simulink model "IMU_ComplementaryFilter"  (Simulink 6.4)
settings: Solver=FixedStepDiscrete  StartTime=0.0  StopTime=10.0  FixedStep=0.001  RelTol=1e-3
undefined symbols (not defined in the file or in its folder): bits, float, gaind, hex2dec, polesd, tustin, zerosd
libraries: dsPICdrivers x31, simulink x13

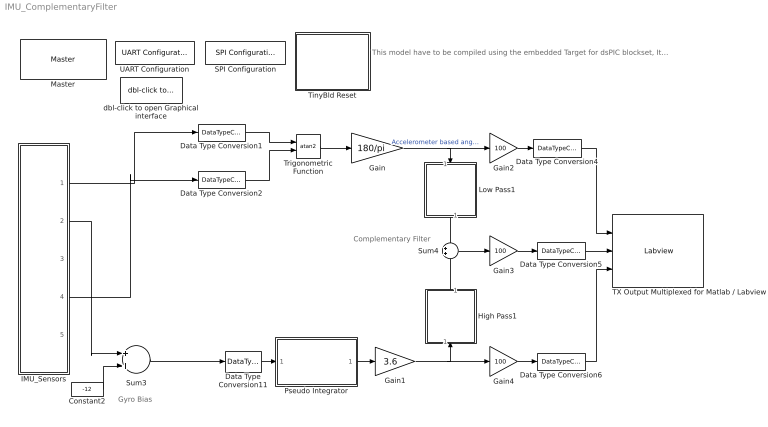
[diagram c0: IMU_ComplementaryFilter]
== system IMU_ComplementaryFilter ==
  note: Gyro Bias
  note: Complementary Filter
  note: This model have to be compiled using the embedded Target for dsPIC blockset, It run on the dsPIC 30f4012 but can be addapted for others MCU.
  Constant2 : Constant  Value=-12  OutDataType=sfix(16)  OutScaling=2^0  SampleTime=-1
  Data Type Conversion1 : DataTypeConversion  OutDataTypeMode=single  OutDataType=sfix(16)  OutScaling="[ (80/(2048*2^4))  0]"
  Data Type Conversion11 : DataTypeConversion  OutDataTypeMode=double  OutDataType=sfix(16)  OutScaling="[ (80/(2048*2^4))  0]"
  Data Type Conversion2 : DataTypeConversion  OutDataTypeMode=single  OutDataType=sfix(16)  OutScaling="[ (80/(2048*2^4))  0]"
  Data Type Conversion4 : DataTypeConversion  OutDataTypeMode=int16  OutDataType=sfix(16)  OutScaling="[ (80/(2048*2^4))  0]"
  Data Type Conversion5 : DataTypeConversion  OutDataTypeMode=int16  OutDataType=sfix(16)  OutScaling="[ (80/(2048*2^4))  0]"
  Data Type Conversion6 : DataTypeConversion  OutDataTypeMode=int16  OutDataType=sfix(16)  OutScaling="[ (80/(2048*2^4))  0]"
  Gain : Gain  Gain=180/pi  ParameterDataType=sfix(16)  ParameterScaling=2^0  OutDataTypeMode=Specify via dialog  OutDataType=float('double')  OutScaling=2^0
  Gain1 : Gain  Gain=3.6  ParameterDataType=sfix(16)  ParameterScaling=2^0  OutDataTypeMode=Specify via dialog  OutDataType=float('double')  OutScaling=2^0
  Gain2 : Gain  Gain=100  ParameterDataType=sfix(16)  ParameterScaling=2^0  OutDataTypeMode=Specify via dialog  OutDataType=float('double')  OutScaling=2^0
  Gain3 : Gain  Gain=100  ParameterDataType=sfix(16)  ParameterScaling=2^0  OutDataTypeMode=Specify via dialog  OutDataType=float('double')  OutScaling=2^0
  Gain4 : Gain  Gain=100  ParameterDataType=sfix(16)  ParameterScaling=2^0  OutDataTypeMode=Specify via dialog  OutDataType=float('double')  OutScaling=2^0
  High Pass1 : Subsystem  Orientation=up  mask(DiscretizedZeroPole){Zeros=[0], Poles=[-.5], Gain=1, AbsTol=auto, SampleTime=.001, method=tustin, Wc=1}
      mask prompts: Zeros "Zeros (enter in s-main:)"; Poles "Poles (enter in s-domain:)"; Gain "Gain (enter in s-domain:)"; AbsTol "Absolute tolerance:"; SampleTime "Sample time:"; Wc "Critical Frequency (Hz):"
      mask help: Continuous mask uses c2d to transform parameters onto the Discrete Zero-Pole block inside.
      mask init:
      | st=SampleTime;
      | if length(st)>1
      |     st=SampleTime(1);
      | end
      | if(st>0)
      |     [zerosd,polesd,gaind] = sldiscutil('disczpk', {st,method,Wc,Zeros,Poles,Gain});
      | end	
      | s = get_param(gcb,'maskvalues');
      | zeross = s{1};
      | poless = s{2};
      | gainss = s{3};
      | %zerosc = eval(zeross);
      | %polesc = eval(poless);
      | %gainsc = eval(gainss);
      | sldiscutil('initzpkmask', st);
      | if(st==0)
      | set_param([gcb '/Zero Pole'], 'AbsoluteTolerance', AbsTol);
      | end
  IMU_Sensors : Subsystem
  Low Pass1 : Subsystem  Orientation=down  mask(DiscretizedZeroPole){Zeros=[], Poles=[-.5], Gain=.5, AbsTol=auto, SampleTime=.001, method=tustin, Wc=1}
      mask prompts: Zeros "Zeros (enter in s-main:)"; Poles "Poles (enter in s-domain:)"; Gain "Gain (enter in s-domain:)"; AbsTol "Absolute tolerance:"; SampleTime "Sample time:"; Wc "Critical Frequency (Hz):"
      mask help: Continuous mask uses c2d to transform parameters onto the Discrete Zero-Pole block inside.
      mask init:
      | st=SampleTime;
      | if length(st)>1
      |     st=SampleTime(1);
      | end
      | if(st>0)
      |     [zerosd,polesd,gaind] = sldiscutil('disczpk', {st,method,Wc,Zeros,Poles,Gain});
      | end	
      | s = get_param(gcb,'maskvalues');
      | zeross = s{1};
      | poless = s{2};
      | gainss = s{3};
      | %zerosc = eval(zeross);
      | %polesc = eval(poless);
      | %gainsc = eval(gainss);
      | sldiscutil('initzpkmask', st);
      | if(st==0)
      | set_param([gcb '/Zero Pole'], 'AbsoluteTolerance', AbsTol);
      | end
  Master : dsPICdrivers/Master  Tag=dsPIC_MASTER  Priority=1  TimeStepType=Timer1  picType=30f4012  fcy=20e6  Quartz_33f=5e6  PLLActive_33f=off  fcyDesired_33f=0  tmr1="[1  19999  0]"  tmr1Info="Time Step : 0.001  ;   Error : 0%  PR1=19999"  tmr2345="[0  0  0  0]"  tmr2345cfg=[-1 -1 -1 -1]  IOautoConf=on  typePort="[ 0   0   0   0   0   0   0   0   0   0   0   0   0   0   0   0   0   0   0   0   0   0   0   0   0   0   0   0   0   0   0   0   0   0   0   0   0   0   0   0   0   0   0   0   0   5   4   0   0   0   0   0   0   0   0   0   0   0   0   0   0   0   0   0   0   0   0  10   0  10   0   0  17   0   0   0   0   0   0   0   0   0  14  15   0   0   0   0   0   0   0   0   0   0   0   0   0   0   0   0 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"  TRIS="[ 65535  65535  65535  65535  65495  65535  65535 ]"  ADPCFG=0  MasterBusyPort=None  MasterOverloadPort=None  FOSC=XT_PLL8  TempProtection_33f=TEMP_ON  FPBOR=PBOR_OFF  PWRT=PWRT_4  MCLR=MCLR_DIS  PowerSave=off
  Pseudo Integrator : Subsystem  mask(DiscretizedZeroPole){Zeros=[0 -314], Poles=[-.03 -.03], Gain=(1/314), AbsTol=auto, SampleTime=.001, method=tustin, Wc=1}
      mask prompts: Zeros "Zeros (enter in s-main:)"; Poles "Poles (enter in s-domain:)"; Gain "Gain (enter in s-domain:)"; AbsTol "Absolute tolerance:"; SampleTime "Sample time:"; Wc "Critical Frequency (Hz):"
      mask help: Continuous mask uses c2d to transform parameters onto the Discrete Zero-Pole block inside.
      mask init:
      | st=SampleTime;
      | if length(st)>1
      |     st=SampleTime(1);
      | end
      | if(st>0)
      |     [zerosd,polesd,gaind] = sldiscutil('disczpk', {st,method,Wc,Zeros,Poles,Gain});
      | end	
      | s = get_param(gcb,'maskvalues');
      | zeross = s{1};
      | poless = s{2};
      | gainss = s{3};
      | %zerosc = eval(zeross);
      | %polesc = eval(poless);
      | %gainsc = eval(gainss);
      | sldiscutil('initzpkmask', st);
      | if(st==0)
      | set_param([gcb '/Zero Pole'], 'AbsoluteTolerance', AbsTol);
      | end
  SPI Configuration : dsPICdrivers/SPI PORT/SPI Configuration  Tag=dsPIC_config_SPI  Priority=2  ConfigurationTime=At boot time (only once)  OrderingInOutPopup=None  SampleTime=-1  Frame_Enable=0  Frame_Sync=0  SPI=1  MODE=MASTER  USER_SCALER=12  StartEnable=Enable  SDO_EN=on  DATA_LENGTH=16 bits  SS_EN=off  SMP=Middle of bit  CKP=high  CKE=Idle to Active  Status="Mode 1  -    Fsck= Not Available"
  Sum3 : Sum  OutDataType=sfix(16)  OutScaling=2^0
  Sum4 : Sum  OutDataType=sfix(16)  OutScaling=2^0
  TX Output Multiplexed for Matlab / Labview : dsPICdrivers/Serial PORT/TX Output Multiplexed for Matlab // Labview  Tag=dsPIC_TX_Multiplexed  Priority=5  UART=1  CleverSpreadingChk=on  CleverSpreading=1  CHANNEL=[0 1 2 ]  BUFFERSIZE=16  CHANNELBLOCKED=[]  CHANNELBLOCKED_BITEWISE=0  Status=OK
  TinyBld Reset : Subsystem  AncestorBlock=dsPICdrivers/OTHERS/TinyBld Reset
  Trigonometric Function : Trigonometry  Operator=atan2  OutputSignalType=real
  UART Configuration : dsPICdrivers/Serial PORT/UART Configuration  Tag=dsPIC_config_UART  Priority=2  UART=1  proposed_BAUD=115200  ALT_TX_RX=on  TXInterruptPri=1  InterruptTxWhen=on TxBUF becoming empty  TXEN=on  RXInterruptPri=1  BAUD=115200  UxBRG=10  Info="UxBRG = 10   ||  Real Baud : 113636   ||  % error : -1.3573  ||  max 11.3636 Bytes / Step"  RealBaud=0
  dbl-click to open Graphical interface : dsPICdrivers/Serial PORT/dbl-click to open Graphical interface  SystemSampleTime=-1
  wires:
  Trigonometric Function/1 -> Gain/1
  Constant2/1 -> Sum3/2
  Low Pass1/1(Out1) -> Sum4/1
  High Pass1/1(Out1) -> Sum4/2
  Pseudo Integrator/1(Out1) -> Gain1/1
  Gain1/1 -> High Pass1/1(In1), Gain4/1
  Gain/1 -> Low Pass1/1(In1), Gain2/1  "Accelerometer based angle estimation"
  Sum4/1 -> Gain3/1
  Data Type Conversion2/1 -> Trigonometric Function/2
  Data Type Conversion1/1 -> Trigonometric Function/1
  Data Type Conversion11/1 -> Pseudo Integrator/1(In1)
  Sum3/1 -> Data Type Conversion11/1
  IMU_Sensors/1(AccelX) -> Data Type Conversion1/1
  IMU_Sensors/4(AccelZ) -> Data Type Conversion2/1
  IMU_Sensors/2(GyroY) -> Sum3/1
  Data Type Conversion4/1 -> TX Output Multiplexed for Matlab / Labview/1
  Gain2/1 -> Data Type Conversion4/1
  Gain3/1 -> Data Type Conversion5/1
  Gain4/1 -> Data Type Conversion6/1
  Data Type Conversion5/1 -> TX Output Multiplexed for Matlab / Labview/2
  Data Type Conversion6/1 -> TX Output Multiplexed for Matlab / Labview/3

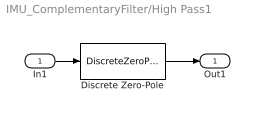
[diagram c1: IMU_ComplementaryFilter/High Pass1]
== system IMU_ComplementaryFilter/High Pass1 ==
  In1 : Inport  OutDataType=sfix(16)  OutScaling=2^0
  Discrete Zero-Pole : DiscreteZeroPole  Zeros=zerosd  Poles=polesd  Gain=gaind  SampleTime=SampleTime
  Out1 : Outport  OutDataType=sfix(16)  OutScaling=2^0
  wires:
  Discrete Zero-Pole/1 -> Out1/1
  In1/1 -> Discrete Zero-Pole/1

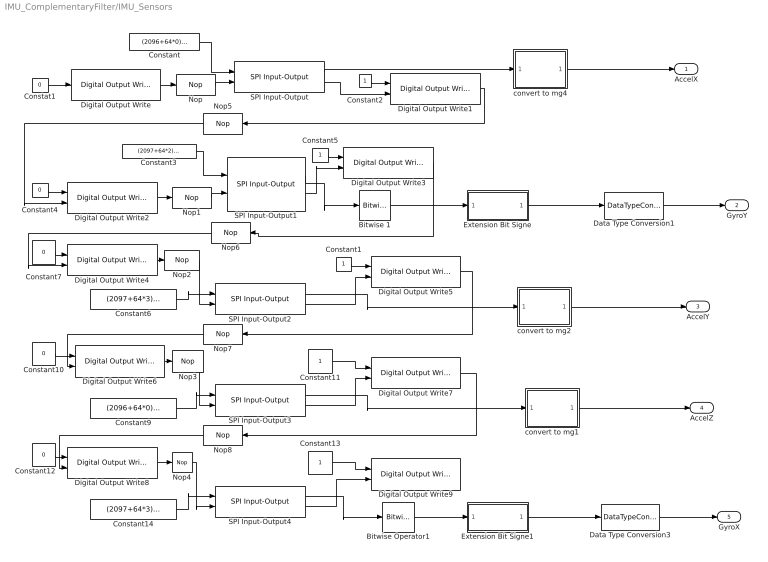
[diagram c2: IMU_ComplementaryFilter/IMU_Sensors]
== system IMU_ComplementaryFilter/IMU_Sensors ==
  Bitwise Operator1 : simulink/Logic and Bit Operations/Bitwise Operator  logicop=AND  UseBitMask=on  BitMask=hex2dec('0FFF')  BitMaskRealWorld=Stored Integer
  Bitwise 1 : simulink/Logic and Bit Operations/Bitwise Operator  logicop=AND  UseBitMask=on  BitMask=hex2dec('0FFF')  BitMaskRealWorld=Stored Integer
  Constant : Constant  Value=(2096+64*0)*16  OutDataTypeMode=uint16  OutDataType=sfix(16)  OutScaling=2^0  SampleTime=-1
  Constant{1..2,5,11,13} (5 alike) : Constant  OutDataTypeMode=boolean  OutDataType=sfix(16)  OutScaling=2^0  SampleTime=-1
  Constant{4,7,10,12} (4 alike) : Constant  Value=0  OutDataTypeMode=boolean  OutDataType=sfix(16)  OutScaling=2^0  SampleTime=-1
  Constant14 : Constant  Value=(2097+64*3)*16  OutDataTypeMode=uint16  OutDataType=sfix(16)  OutScaling=2^0  SampleTime=-1
  Constant3 : Constant  Value=(2097+64*2)*16  VectorParams1D=off  OutDataTypeMode=uint16  OutDataType=sfix(16)  OutScaling=2^0  SampleTime=-1
  Constant6 : Constant  Value=(2097+64*3)*16  OutDataTypeMode=uint16  OutDataType=sfix(16)  OutScaling=2^0  SampleTime=-1
  Constant9 : Constant  Value=(2096+64*0)*16  OutDataTypeMode=uint16  OutDataType=sfix(16)  OutScaling=2^0  SampleTime=-1
  Constat1 : Constant  Value=0  OutDataTypeMode=boolean  OutDataType=sfix(16)  OutScaling=2^0  SampleTime=-1
  Data Type Conversion1 : DataTypeConversion  OutDataTypeMode=Specify via dialog  OutDataType=sfix(12)  OutScaling="[ (160/4096)  0]"  ConvertRealWorld=Stored Integer (SI)
  Data Type Conversion3 : DataTypeConversion  OutDataTypeMode=Specify via dialog  OutDataType=sfix(12)  OutScaling="[ (160/4096)  0]"  ConvertRealWorld=Stored Integer (SI)
  Digital Output Write : dsPICdrivers/Digital I//O/Digital Output Write  Tag=dsPIC_Digital_Output  Priority=5  PORT=E  Pin=5  Simultaneous=off  OrderingInOutPopup=Output
  Digital Output Write{1..5} (5 alike) : dsPICdrivers/Digital I//O/Digital Output Write  Tag=dsPIC_Digital_Output  Priority=5  PORT=E  Pin=5  Simultaneous=off  OrderingInOutPopup=Input & Output
  Digital Output Write6 : dsPICdrivers/Digital I//O/Digital Output Write  Tag=dsPIC_Digital_Output  Priority=5  PORT=E  Pin=3  Simultaneous=off  OrderingInOutPopup=Input & Output
  Digital Output Write7 : dsPICdrivers/Digital I//O/Digital Output Write  Tag=dsPIC_Digital_Output  Priority=5  PORT=E  Pin=3  Simultaneous=off  OrderingInOutPopup=Input & Output
  Digital Output Write8 : dsPICdrivers/Digital I//O/Digital Output Write  Tag=dsPIC_Digital_Output  Priority=5  PORT=E  Pin=3  Simultaneous=off  OrderingInOutPopup=Input & Output
  Digital Output Write9 : dsPICdrivers/Digital I//O/Digital Output Write  Tag=dsPIC_Digital_Output  Priority=5  PORT=E  Pin=3  Simultaneous=off  OrderingInOutPopup=Input
  Extension Bit Signe : Subsystem  TreatAsAtomicUnit=on
  Extension Bit Signe1 : Subsystem  TreatAsAtomicUnit=on
  Nop{,1..4} (5 alike) : dsPICdrivers/OTHERS/Nop  Tag=dsPIC_Reset  NbrNop=5
  Nop{5..8} (4 alike) : dsPICdrivers/OTHERS/Nop  Tag=dsPIC_Reset  Orientation=left  NbrNop=5
  SPI Input-Output{,1..4} (5 alike) : dsPICdrivers/SPI PORT/SPI Input-Output  Tag=dsPIC_SPI  SPI=1  INPUT=on  RESET_INPUT=off  OUTPUT=on  SPECIAL_SPI=Always Enable  DATA_LENGTH=16 bits  WAIT_INPUTDATA=on  OrderingInOutPopup=Input & Output  SampleTime=-1
  convert to mg1 : Subsystem  TreatAsAtomicUnit=on
  convert to mg2 : Subsystem  TreatAsAtomicUnit=on
  convert to mg4 : Subsystem  TreatAsAtomicUnit=on
  AccelX : Outport  OutDataType=sfix(16)  OutScaling=2^0
  GyroY : Outport  Port=2  OutDataType=sfix(16)  OutScaling=2^0
  AccelY : Outport  Port=3  OutDataType=sfix(16)  OutScaling=2^0
  AccelZ : Outport  Port=4  OutDataType=sfix(16)  OutScaling=2^0
  GyroX : Outport  Port=5  OutDataType=sfix(16)  OutScaling=2^0
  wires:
  Extension Bit Signe1/1(Out1) -> Data Type Conversion3/1
  Extension Bit Signe/1(Out1) -> Data Type Conversion1/1
  Bitwise 1/1 -> Extension Bit Signe/1(In1)
  Digital Output Write3/1 -> Nop6/1
  convert to mg2/1(Out1) -> AccelY/1
  convert to mg1/1(Out1) -> AccelZ/1
  Data Type Conversion3/1 -> GyroX/1
  Bitwise Operator1/1 -> Extension Bit Signe1/1(In1)
  Nop8/1 -> Digital Output Write8/2
  Nop7/1 -> Digital Output Write6/2
  Nop6/1 -> Digital Output Write4/2
  Nop5/1 -> Digital Output Write2/2
  Nop4/1 -> SPI Input-Output4/2
  Nop3/1 -> SPI Input-Output3/2
  Nop2/1 -> SPI Input-Output2/2
  Nop1/1 -> SPI Input-Output1/2
  Nop/1 -> SPI Input-Output/2
  Data Type Conversion1/1 -> GyroY/1
  convert to mg4/1(Out1) -> AccelX/1
  SPI Input-Output4/2 -> Digital Output Write9/2
  SPI Input-Output4/1 -> Bitwise Operator1/1
  Digital Output Write8/1 -> Nop4/1
  Constant14/1 -> SPI Input-Output4/1
  SPI Input-Output3/2 -> Digital Output Write7/2
  SPI Input-Output3/1 -> convert to mg1/1(In1)
  Constant9/1 -> SPI Input-Output3/1
  Digital Output Write6/1 -> Nop3/1
  SPI Input-Output2/2 -> Digital Output Write5/2
  SPI Input-Output2/1 -> convert to mg2/1(In1)
  Constant6/1 -> SPI Input-Output2/1
  Digital Output Write4/1 -> Nop2/1
  Constant7/1 -> Digital Output Write4/1
  SPI Input-Output1/1 -> Bitwise 1/1
  SPI Input-Output1/2 -> Digital Output Write3/2
  Digital Output Write2/1 -> Nop1/1
  Constant3/1 -> SPI Input-Output1/1
  SPI Input-Output/1 -> convert to mg4/1(In1)
  SPI Input-Output/2 -> Digital Output Write1/2
  Constant/1 -> SPI Input-Output/1
  Digital Output Write/1 -> Nop/1
  Digital Output Write7/1 -> Nop8/1
  Constant12/1 -> Digital Output Write8/1
  Constant13/1 -> Digital Output Write9/1
  Digital Output Write5/1 -> Nop7/1
  Constant10/1 -> Digital Output Write6/1
  Constant11/1 -> Digital Output Write7/1
  Constant1/1 -> Digital Output Write5/1
  Digital Output Write1/1 -> Nop5/1
  Constant4/1 -> Digital Output Write2/1
  Constant5/1 -> Digital Output Write3/1
  Constat1/1 -> Digital Output Write/1
  Constant2/1 -> Digital Output Write1/1

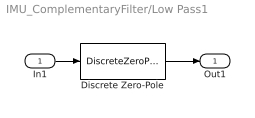
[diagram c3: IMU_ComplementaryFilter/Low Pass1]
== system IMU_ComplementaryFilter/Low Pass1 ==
  In1 : Inport  OutDataType=sfix(16)  OutScaling=2^0
  Discrete Zero-Pole : DiscreteZeroPole  Zeros=zerosd  Poles=polesd  Gain=gaind  SampleTime=SampleTime
  Out1 : Outport  OutDataType=sfix(16)  OutScaling=2^0
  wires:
  In1/1 -> Discrete Zero-Pole/1
  Discrete Zero-Pole/1 -> Out1/1

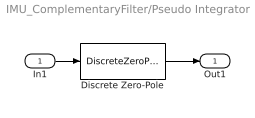
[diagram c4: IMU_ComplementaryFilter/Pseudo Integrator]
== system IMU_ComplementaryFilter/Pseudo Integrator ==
  In1 : Inport  OutDataType=sfix(16)  OutScaling=2^0
  Discrete Zero-Pole : DiscreteZeroPole  Zeros=zerosd  Poles=polesd  Gain=gaind  SampleTime=SampleTime
  Out1 : Outport  OutDataType=sfix(16)  OutScaling=2^0
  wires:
  Discrete Zero-Pole/1 -> Out1/1
  In1/1 -> Discrete Zero-Pole/1

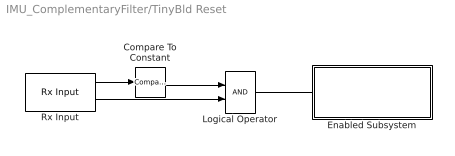
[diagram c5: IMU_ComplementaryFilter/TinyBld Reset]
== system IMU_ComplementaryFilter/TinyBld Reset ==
  Compare To Constant : simulink/Logic and Bit Operations/Compare To Constant  SystemSampleTime=-1  relop===  const=55  LogicOutDataTypeMode=boolean  ZeroCross=off
  Enabled Subsystem : Subsystem  Orientation=up  TreatAsAtomicUnit=on
  Logical Operator : Logic  AllPortsSameDT=off  OutDataTypeMode=boolean
  Rx Input : dsPICdrivers/Serial PORT/Rx Input  Tag=dsPIC_RX  Priority=5  UART=1  SampleTime=.01  BlockingFctChk=off  OutputDefault=0  IsPresentFlagChk=on
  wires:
  Rx Input/1 -> Compare To Constant/1
  Compare To Constant/1 -> Logical Operator/1
  Rx Input/2 -> Logical Operator/2
  Logical Operator/1 -> Enabled Subsystem/Enable

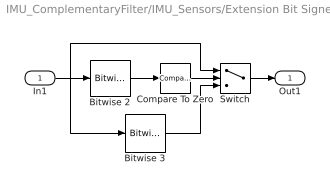
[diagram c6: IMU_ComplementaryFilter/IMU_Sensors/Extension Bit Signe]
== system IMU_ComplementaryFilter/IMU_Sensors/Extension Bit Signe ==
  In1 : Inport  OutDataType=sfix(16)  OutScaling=2^0
  Bitwise 2 : simulink/Logic and Bit Operations/Bitwise Operator  logicop=AND  UseBitMask=on  BitMask=2^11  BitMaskRealWorld=Stored Integer
  Bitwise 3 : simulink/Logic and Bit Operations/Bitwise Operator  logicop=OR  UseBitMask=on  BitMask=hex2dec('F000')  BitMaskRealWorld=Stored Integer
  Compare To Zero : simulink/Logic and Bit Operations/Compare To Zero  SystemSampleTime=-1  relop===  LogicOutDataTypeMode=boolean  ZeroCross=off
  Switch : Switch  Criteria=u2 ~= 0
  Out1 : Outport  OutDataType=sfix(16)  OutScaling=2^0
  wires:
  Switch/1 -> Out1/1
  Bitwise 3/1 -> Switch/3
  Compare To Zero/1 -> Switch/2
  Bitwise 2/1 -> Compare To Zero/1
  In1/1 -> Bitwise 2/1, Switch/1, Bitwise 3/1

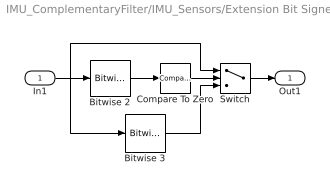
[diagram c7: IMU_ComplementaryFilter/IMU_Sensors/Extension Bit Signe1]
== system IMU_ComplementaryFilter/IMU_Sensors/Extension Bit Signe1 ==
  In1 : Inport  OutDataType=sfix(16)  OutScaling=2^0
  Bitwise 2 : simulink/Logic and Bit Operations/Bitwise Operator  logicop=AND  UseBitMask=on  BitMask=2^11  BitMaskRealWorld=Stored Integer
  Bitwise 3 : simulink/Logic and Bit Operations/Bitwise Operator  logicop=OR  UseBitMask=on  BitMask=hex2dec('F000')  BitMaskRealWorld=Stored Integer
  Compare To Zero : simulink/Logic and Bit Operations/Compare To Zero  SystemSampleTime=-1  relop===  LogicOutDataTypeMode=boolean  ZeroCross=off
  Switch : Switch  Criteria=u2 ~= 0
  Out1 : Outport  OutDataType=sfix(16)  OutScaling=2^0
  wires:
  In1/1 -> Bitwise 3/1, Switch/1, Bitwise 2/1
  Bitwise 2/1 -> Compare To Zero/1
  Compare To Zero/1 -> Switch/2
  Bitwise 3/1 -> Switch/3
  Switch/1 -> Out1/1

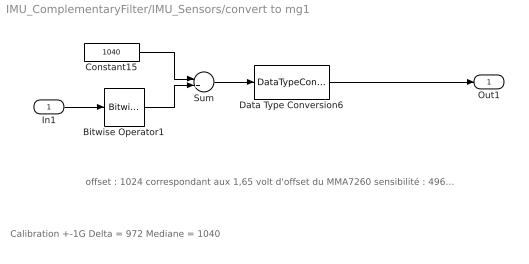
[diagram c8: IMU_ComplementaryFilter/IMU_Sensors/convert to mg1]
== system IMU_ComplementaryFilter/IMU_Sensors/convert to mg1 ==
  note: Calibration +-1G Delta = 972 Mediane = 1040
  note: offset : 1024 correspondant aux 1,65 volt d'offset du MMA7260 sensibilité : 496.484848 / g ==> (2mg) Le composant est alimenté en 2.5V au lieu de 3.3V
  In1 : Inport  OutDataType=sfix(16)  OutScaling=2^0
  Bitwise Operator1 : simulink/Logic and Bit Operations/Bitwise Operator  logicop=AND  UseBitMask=on  BitMask=4095  BitMaskRealWorld=Stored Integer
  Constant15 : Constant  Value=1040  OutDataTypeMode=int16  OutDataType=sfix(16)  OutScaling=2^0  SampleTime=-1
  Data Type Conversion6 : DataTypeConversion  OutDataTypeMode=Specify via dialog  OutDataType=sfix(12)  OutScaling=[1/486*1000 0]  ConvertRealWorld=Stored Integer (SI)
  Sum : Sum  Inputs=-+  OutDataTypeMode=int16  OutDataType=sfix(16)  OutScaling=2^0
  Out1 : Outport  OutDataType=sfix(16)  OutScaling=2^0
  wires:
  Bitwise Operator1/1 -> Sum/2
  Sum/1 -> Data Type Conversion6/1
  Constant15/1 -> Sum/1
  Data Type Conversion6/1 -> Out1/1
  In1/1 -> Bitwise Operator1/1

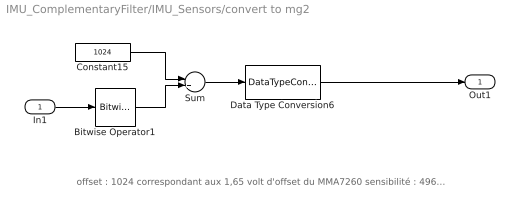
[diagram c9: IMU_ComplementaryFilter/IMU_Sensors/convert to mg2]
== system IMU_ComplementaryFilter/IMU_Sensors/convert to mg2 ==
  note: offset : 1024 correspondant aux 1,65 volt d'offset du MMA7260 sensibilité : 496.484848 / g ==> (2mg) Le composant est alimenté en 2.5V au lieu de 3.3V
  In1 : Inport  OutDataType=sfix(16)  OutScaling=2^0
  Bitwise Operator1 : simulink/Logic and Bit Operations/Bitwise Operator  logicop=AND  UseBitMask=on  BitMask=4095  BitMaskRealWorld=Stored Integer
  Constant15 : Constant  Value=1024  OutDataTypeMode=int16  OutDataType=sfix(16)  OutScaling=2^0  SampleTime=-1
  Data Type Conversion6 : DataTypeConversion  OutDataTypeMode=Specify via dialog  OutDataType=sfix(12)  OutScaling=[1/496.484848*1000 0]  ConvertRealWorld=Stored Integer (SI)
  Sum : Sum  Inputs=-+  OutDataTypeMode=int16  OutDataType=sfix(16)  OutScaling=2^0
  Out1 : Outport  OutDataType=sfix(16)  OutScaling=2^0
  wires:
  In1/1 -> Bitwise Operator1/1
  Data Type Conversion6/1 -> Out1/1
  Constant15/1 -> Sum/1
  Sum/1 -> Data Type Conversion6/1
  Bitwise Operator1/1 -> Sum/2

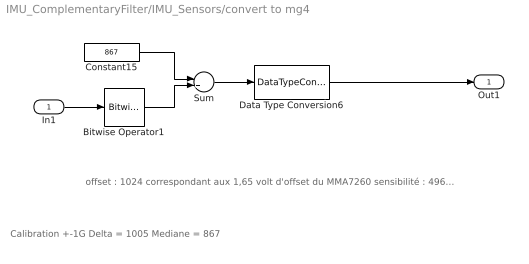
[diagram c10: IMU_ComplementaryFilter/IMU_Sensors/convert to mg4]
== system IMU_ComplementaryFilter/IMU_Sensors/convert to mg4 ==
  note: offset : 1024 correspondant aux 1,65 volt d'offset du MMA7260 sensibilité : 496.484848 / g ==> (2mg) Le composant est alimenté en 2.5V au lieu de 3.3V
  note: Calibration +-1G Delta = 1005 Mediane = 867
  In1 : Inport  OutDataType=sfix(16)  OutScaling=2^0
  Bitwise Operator1 : simulink/Logic and Bit Operations/Bitwise Operator  logicop=AND  UseBitMask=on  BitMask=4095  BitMaskRealWorld=Stored Integer
  Constant15 : Constant  Value=867  OutDataTypeMode=int16  OutDataType=sfix(16)  OutScaling=2^0  SampleTime=-1
  Data Type Conversion6 : DataTypeConversion  OutDataTypeMode=Specify via dialog  OutDataType=sfix(12)  OutScaling=[1/502.5*1000 0]  ConvertRealWorld=Stored Integer (SI)
  Sum : Sum  Inputs=-+  OutDataTypeMode=int16  OutDataType=sfix(16)  OutScaling=2^0
  Out1 : Outport  OutDataType=sfix(16)  OutScaling=2^0
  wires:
  In1/1 -> Bitwise Operator1/1
  Data Type Conversion6/1 -> Out1/1
  Constant15/1 -> Sum/1
  Sum/1 -> Data Type Conversion6/1
  Bitwise Operator1/1 -> Sum/2

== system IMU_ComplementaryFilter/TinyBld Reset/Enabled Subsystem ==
  Enable : EnablePort
  While Iterator Subsystem : Subsystem  TreatAsAtomicUnit=on

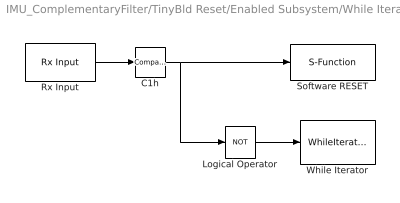
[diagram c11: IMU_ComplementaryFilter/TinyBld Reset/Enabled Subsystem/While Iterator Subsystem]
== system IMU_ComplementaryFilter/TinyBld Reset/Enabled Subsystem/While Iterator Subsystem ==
  C1h : simulink/Logic and Bit Operations/Compare To Constant  SystemSampleTime=-1  relop===  const=66  LogicOutDataTypeMode=boolean  ZeroCross=off
  Logical Operator : Logic  Operator=NOT  AllPortsSameDT=off  OutDataTypeMode=boolean
  Rx Input : dsPICdrivers/Serial PORT/Rx Input  Tag=dsPIC_RX  Priority=5  UART=1  SampleTime=-1  BlockingFctChk=on  OutputDefault=0  IsPresentFlagChk=off
  Software RESET : S-Function  Tag=dsPIC_Reset  FunctionName=dsPIC_Reset
  While Iterator : WhileIterator  MaxIters=-1  WhileBlockType=do-while  ResetStates=reset
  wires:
  Logical Operator/1 -> While Iterator/1
  Rx Input/1 -> C1h/1
  C1h/1 -> Software RESET/1, Logical Operator/1
